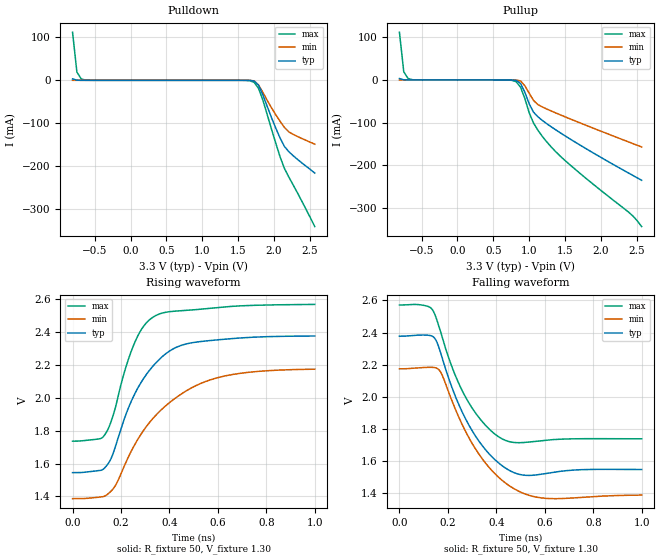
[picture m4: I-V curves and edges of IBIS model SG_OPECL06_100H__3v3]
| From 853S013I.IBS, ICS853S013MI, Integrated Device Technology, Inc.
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[Model] SG_OPECL06_100H__3v3
Model_type   Output_ECL
Polarity   Non-Inverting
|   typ   min   max
C_comp   2pF   1.5pF   2.5pF
Vmeas = 1.97V
Rref = 50
Cref = 0
Vref = 1.3V
|   typ   min   max
[Voltage range]   3.3V   3.135V   3.465V
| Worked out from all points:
|   rising waveform, R_fixture 50, V_fixture 1.30: 20-80 % time 164ps typ, 240ps min, 109ps max; typ from 1.54 V to 2.38 V
|   falling waveform, R_fixture 50, V_fixture 1.30: 20-80 % time 151ps typ, 173ps min, 141ps max; typ from 2.38 V to 1.55 V
[Pulldown]
|Voltage   I (typ)   I (min)   I (max)
|Note, modeling breaks down at 250mA and above.  This is well beyond the functional   |
|operating range of the device.  Should this scenario occur, catastrophic failure and   |
|possible damage to the device and/or board is of higher concern than the I-V curve   |
|behavior.  The IBIS checker will flag currents in excess of 10A with warnings.  Lines   |
|with currents in excess of 0.35 A have been commented out.  The points still remain|
|available to the user if the user desires to use them.   |
|-2.53333e+00   1.36175e+08   1.79237e+08   9.77645e+07
|-1.76667e+00   5.02770e+07   6.93920e+07   3.34409e+07
|-1.00000e+00   5.63549e+00   1.05412e+00   2.60079e+01
|-9.90000e-01   3.82790e+00   6.40804e-01   1.98508e+01
|-9.29670e-01   3.65720e-01   3.18126e-02   3.77220e+00
|-8.69341e-01   3.49411e-02   1.57933e-03   6.50010e-01
-809mV    3.338mA    78.41uA    112mA
-748.7mV  318.9uA    3.892uA    19.3mA
-688.4mV  30.47uA    193.3nA    3.326mA
-567.7mV  278.2nA    509.6pA    98.77uA
1.604V    -19.81uA   -4.568uA   -177.3uA
1.725V    -1.838mA   -1.469mA   -4.916mA
1.785V    -11.51mA   -10.83mA   -18.87mA
1.845V    -33.86mA   -28.1mA    -46.18mA
2.026V    -111.9mA   -80.61mA   -147mA
2.147V    -154.5mA   -110.1mA   -205.7mA
2.268V    -175.8mA   -126mA     -243.9mA
2.569V    -216.4mA   -149mA     -341.1mA
| 2.62978e+00   -2.25125e-01   -1.53511e-01   -3.63426e-01
| 2.69011e+00   -2.34461e-01   -1.58103e-01   -3.82062e-01
| 2.75044e+00   -2.44191e-01   -1.62733e-01   -3.96933e-01
| 2.81077e+00   -2.53841e-01   -1.67437e-01   -4.10969e-01
| 2.87110e+00   -2.64032e-01   -1.72245e-01   -4.24985e-01
| 2.93143e+00   -2.74703e-01   -1.77122e-01   -4.39112e-01
| 2.99176e+00   -2.85550e-01   -1.81866e-01   -4.53233e-01
| 3.05209e+00   -2.97087e-01   -1.86691e-01   -4.66749e-01
| 3.11242e+00   -3.08243e-01   -1.92034e-01   -4.79628e-01
| 3.17275e+00   -3.17584e-01   -1.97628e-01   -4.92057e-01
| 3.23308e+00   -3.26124e-01   -2.03167e-01   -5.04126e-01
| 3.29341e+00   -3.34457e-01   -2.08338e-01   -5.15890e-01
| 3.35374e+00   -3.42724e-01   -2.12844e-01   -5.27385e-01
| 3.41407e+00   -3.50880e-01   -2.16967e-01   -5.38637e-01
| 3.47440e+00   -3.58633e-01   -2.21016e-01   -5.49670e-01
| 3.53473e+00   -3.66005e-01   -2.25042e-01   -5.60503e-01
| 3.59505e+00   -3.73146e-01   -2.29069e-01   -5.71151e-01
| 3.65538e+00   -3.80099e-01   -2.33198e-01   -5.81632e-01
| 3.71571e+00   -3.86892e-01   -2.37691e-01   -5.91965e-01
| 3.77604e+00   -3.93606e-01   -2.42736e-01   -6.02214e-01
| 3.83637e+00   -4.00478e-01   -2.48534e-01   -6.12659e-01
| 3.89670e+00   -4.08266e-01   -2.59800e-01   -6.24776e-01
| 3.95703e+00   -4.23435e-01   -3.73106e-01   -6.46706e-01
| 4.01736e+00   -5.13391e-01   -2.53482e+00   -7.25132e-01
| 4.07769e+00   -1.38387e+00   -3.33694e+01   -1.13069e+00
| 4.13802e+00   -9.11780e+00   -5.96914e+02   -3.43397e+00
| 4.19835e+00   -7.20553e+01   -1.18873e+04   -1.37384e+01
| 4.25868e+00   -7.08149e+02   -2.39207e+05   -6.49500e+01
| 4.31901e+00   -7.34272e+03   -1.39403e+06   -3.53499e+02
| 4.37934e+00   -7.67473e+04   -2.73645e+06   -2.01939e+03
| 4.43967e+00   -6.76901e+05   -6.96606e+06   -1.16775e+04
| 4.50000e+00   -1.61768e+06   -1.68005e+07   -6.77104e+04
| 4.51000e+00   -1.77713e+06   -1.84306e+07   -9.06182e+04
| 5.20667e+00   -7.84755e+07   -1.31996e+08   -3.92054e+07
| 5.90333e+00   -1.67282e+08   -2.45561e+08   -1.05707e+08
| 6.60000e+00   -2.56089e+08   -3.59126e+08   -1.72209e+08
[Pullup]
|Voltage   I (typ)   I (min)   I (max)
|Note, modeling breaks down at 250mA and above.  This is well beyond the functional   |
|operating range of the device.  Should this scenario occur, catastrophic failure and   |
|possible damage to the device and/or board is of higher concern than the I-V curve   |
|behavior.  The IBIS checker will flag currents in excess of 10A with warnings.  Lines   |
|with currents in excess of 0.35 A have been commented out.  The points still remain|
|available to the user if the user desires to use them.   |
|-2.53333e+00   1.36175e+08   1.79237e+08   9.77645e+07
|-1.76667e+00   5.02770e+07   6.93920e+07   3.34409e+07
|-1.00000e+00   5.63549e+00   1.05412e+00   2.60079e+01
|-9.90000e-01   3.82790e+00   6.40804e-01   1.98508e+01
|-9.29670e-01   3.65720e-01   3.18126e-02   3.77220e+00
|-8.69341e-01   3.49411e-02   1.57933e-03   6.50010e-01
-809mV    3.338mA    78.41uA    112mA
-748.7mV  318.9uA    3.892uA    19.3mA
-688.4mV  30.47uA    193.3nA    3.326mA
699.2mV   -11.98uA   -403.3nA   -150.5uA
819.9mV   -1.151mA   -147.8uA   -4.251mA
880.2mV   -8.303mA   -2.318mA   -17.02mA
1.001V    -56.04mA   -31.17mA   -77.13mA
1.061V    -75.64mA   -48mA      -101.2mA
1.242V    -102.4mA   -68mA      -144.7mA
1.604V    -142.2mA   -93.71mA   -204.4mA
2.388V    -218.9mA   -145.7mA   -310.8mA
2.569V    -235.8mA   -157.5mA   -344.5mA
| 2.62978e+00   -2.41325e-01   -1.61350e-01   -3.59600e-01
| 2.69011e+00   -2.46882e-01   -1.65242e-01   -3.75753e-01
| 2.75044e+00   -2.52475e-01   -1.69130e-01   -3.92180e-01
| 2.81077e+00   -2.58322e-01   -1.73038e-01   -4.08288e-01
| 2.87110e+00   -2.64987e-01   -1.76987e-01   -4.23986e-01
| 2.93143e+00   -2.72998e-01   -1.80957e-01   -4.39114e-01
| 2.99176e+00   -2.82248e-01   -1.84931e-01   -4.53204e-01
| 3.05209e+00   -2.92183e-01   -1.88917e-01   -4.66556e-01
| 3.11242e+00   -3.02397e-01   -1.93042e-01   -4.79391e-01
| 3.17275e+00   -3.12680e-01   -1.97483e-01   -4.91816e-01
| 3.23308e+00   -3.22893e-01   -2.02134e-01   -5.03893e-01
| 3.29341e+00   -3.32384e-01   -2.06860e-01   -5.15665e-01
| 3.35374e+00   -3.40743e-01   -2.11579e-01   -5.27168e-01
| 3.41407e+00   -3.48522e-01   -2.16195e-01   -5.38428e-01
| 3.47440e+00   -3.55948e-01   -2.20410e-01   -5.49468e-01
| 3.53473e+00   -3.63122e-01   -2.24515e-01   -5.60305e-01
| 3.59505e+00   -3.70098e-01   -2.28594e-01   -5.70958e-01
| 3.65538e+00   -3.76917e-01   -2.32763e-01   -5.81441e-01
| 3.71571e+00   -3.83625e-01   -2.37287e-01   -5.91775e-01
| 3.77604e+00   -3.90337e-01   -2.42362e-01   -6.02023e-01
| 3.83637e+00   -3.97300e-01   -2.48190e-01   -6.12467e-01
| 3.89670e+00   -4.05262e-01   -2.59490e-01   -6.24581e-01
| 3.95703e+00   -4.20660e-01   -3.72830e-01   -6.46506e-01
| 4.01736e+00   -5.10881e-01   -2.53458e+00   -7.24925e-01
| 4.07769e+00   -1.38164e+00   -3.33692e+01   -1.13047e+00
| 4.13802e+00   -9.11580e+00   -5.96914e+02   -3.43374e+00
| 4.19835e+00   -7.20535e+01   -1.18873e+04   -1.37382e+01
| 4.25868e+00   -7.08147e+02   -2.39207e+05   -6.49498e+01
| 4.31901e+00   -7.34272e+03   -1.39403e+06   -3.53499e+02
| 4.37934e+00   -7.67473e+04   -2.73645e+06   -2.01939e+03
| 4.43967e+00   -6.76901e+05   -6.96606e+06   -1.16775e+04
| 4.50000e+00   -1.61768e+06   -1.68005e+07   -6.77104e+04
| 4.51000e+00   -1.77713e+06   -1.84306e+07   -9.06182e+04
| 5.20667e+00   -7.84755e+07   -1.31996e+08   -3.92054e+07
| 5.90333e+00   -1.67282e+08   -2.45561e+08   -1.05707e+08
| 6.60000e+00   -2.56089e+08   -3.59126e+08   -1.72209e+08
[Ramp]
|   typ   min   max
dV/dt_r   0.498/0.163n   0.472/0.24n   0.499/0.109n
dV/dt_f   0.525/0.164n   0.491/0.183n   0.517/0.15n
R_load =   50.0000
[Rising Waveform]
R_fixture = 50
V_fixture = 1.30   | VCC_typ - 2V
V_fixture_max = 1.465   | VCC_max - 2V
V_fixture_min = 1.135   | VCC_min - 2V
C_fixture = 0.0p
| Time   typ   min   max
0s        1.545V     1.387V     1.736V
135.1ps   1.578V     1.404V     1.78V
178.2ps   1.71V      1.47V      1.948V
214.2ps   1.875V     1.587V     2.158V
253.3ps   2.013V     1.706V     2.324V
292.3ps   2.116V     1.8V       2.434V
338.3ps   2.204V     1.885V     2.496V
435.4ps   2.312V     2.01V      2.529V
582.6ps   2.351V     2.116V     2.547V
1ns       2.376V     2.174V     2.568V
[Falling Waveform]
R_fixture = 50
V_fixture = 1.30   | VCC_typ - 2V
V_fixture_max = 1.465   | VCC_max - 2V
V_fixture_min = 1.135   | VCC_min - 2V
C_fixture = 0.0p
| Time   typ   min   max
0s        2.377V     2.174V     2.572V
110.1ps   2.384V     2.183V     2.567V
145.1ps   2.365V     2.182V     2.517V
174.2ps   2.253V     2.142V     2.385V
269.3ps   1.873V     1.795V     2.008V
340.3ps   1.698V     1.616V     1.848V
420.4ps   1.574V     1.483V     1.74V
498.5ps   1.515V     1.407V     1.714V
590.6ps   1.518V     1.369V     1.727V
1ns       1.546V     1.387V     1.738V
